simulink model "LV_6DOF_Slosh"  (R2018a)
settings: Solver=FixedStepAuto  StartTime=0.0  StopTime=489.8  FixedStep=0.0002  MaxStep=0.0001  RelTol=2e-6  EnableMultiTasking=on
InitFcn:
  | init
StopFcn:
  | pl
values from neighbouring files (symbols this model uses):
  accel = [97.3083,0,0]    [init.m]
  AcNoise = 0.1    [init.m]
  BBrcs = [82, 0.0, +3.375]    [init.m]
  Cdelay = 0.005    [init.m]
  Cza1 = FCS_Gains_Stg1(:, 5)    [init.m]
  d2r = pi/180    (= 0.0174532925199)    [init.m]    (also in pl.m; LQR_Design.m)
  Euler_0 = [90, 89.98, 0]*d2r    [init.m]
  fairing_mass = 1047.7*kg2slug    (= 71.7904994)    [init.m]
  Ie1 = 28.17    [init.m]
  Ie2 = 258.74    [init.m]
  Islosh = 1    [init.m]
  Isp = 65    [init.m]
  Ixxpr = Mass_Props(:,2)    [init.m]
  Ixypr = Mass_Props(:,5)    [init.m]
  Ixzpr = Mass_Props(:,6)    [init.m]
  Iyypr = Mass_Props(:,3)    [init.m]
  Iyzpr = Mass_Props(:,7)    [init.m]
  Izzpr = Mass_Props(:,4)    [init.m]
  Jdir = zeros(3,nt)    [init.m]
  JJ1 = Commands_2(:,2)    [init.m]
  JJ2 = Commands_2(:,3)    [init.m]
  JJ3 = Commands_2(:,4)    [init.m]
  Jloc = Jdir    [init.m]
  K_estim1 = FCS_Gains_Stg1(:,21)    [init.m]
  Kl_p1 = FCS_Gains_Stg1(:,12)    [init.m]
  Kl_phi1 = FCS_Gains_Stg1(:,11)    [init.m]
  Km_alfa1 = FCS_Gains_Stg1(:, 8)    [init.m]
  Km_alfin = FCS_Gains_Stg1(:,10)    [init.m]
  Km_q1 = FCS_Gains_Stg1(:, 7)    [init.m]
  Km_q2 = FCS_Gains_Stg2(:,5)    [init.m]
  Km_thet1 = FCS_Gains_Stg1(:, 6)    [init.m]
  Km_thet2 = FCS_Gains_Stg2(:,4)    [init.m]
  Km_thin1 = FCS_Gains_Stg1(:, 9)    [init.m]
  Km_thin2 = FCS_Gains_Stg2(:,6)    [init.m]
  Kmix2 = [ 0,   -1,    0;          0,    0,   -1]    [init.m]
  Kml1_1 = ee*FCS_Gains_Stg1(:,18)    [init.m]
  Kml2_1 = ee*FCS_Gains_Stg1(:,19)    [init.m]
  Kml2_2 = ee*FCS_Gains_Stg2(:,10)    [init.m]
  Kn_beta1 = FCS_Gains_Stg1(:,15)    [init.m]
  Kn_betin = FCS_Gains_Stg1(:,17)    [init.m]
  Kn_psi1 = FCS_Gains_Stg1(:,13)    [init.m]
  Kn_psi2 = FCS_Gains_Stg2(:,7)    [init.m]
  Kn_psin1 = FCS_Gains_Stg1(:,16)    [init.m]
  Kn_psin2 = FCS_Gains_Stg2(:,9)    [init.m]
  Kn_r1 = FCS_Gains_Stg1(:,14)    [init.m]
  Kn_r2 = FCS_Gains_Stg2(:,8)    [init.m]
  Le1 = 1.203    [init.m]
  Le2 = 2.892    [init.m]
  Massgn1 = ee*FCS_Gains_Stg1(:,2)    [init.m]
  Massgn2 = ee*FCS_Gains_Stg2(:,2)    [init.m]
  mdot1 = 2.5058    [init.m]
  mdot2 = 2.5058    [init.m]
  me1 = 9.325    [init.m]
  me2 = 13.927    [init.m]
  mrc = [x_ref, y_ref, z_ref]    [init.m]
  Msfue = Slosh(:,3)    [init.m]
  Mslox = Slosh(:,2)    [init.m]
  msspr = Mass_Props(:,1)    [init.m]
  Mvsls = Slosh(:,1)    [init.m]
  post_sep_wait = 4    [init.m]
  pre_sep_wait = 4    [init.m]
  Qbar1 = FCS_Gains_Stg1(:, 4)    [init.m]
  qtc1 = interp1(timi2(1:iend),Commands_2(1:iend, 9),timi2,'linear','extrap')    [init.m]
  qtc2 = interp1(timi2(1:iend),Commands_2(1:iend,10),timi2,'linear','extrap')    [init.m]
  qtc3 = interp1(timi2(1:iend),Commands_2(1:iend,11),timi2,'linear','extrap')    [init.m]
  qtc4 = interp1(timi2(1:iend),Commands_2(1:iend,12),timi2,'linear','extrap')    [init.m]
  r2d = 1/d2r    (= 57.2957795131)    [init.m]    (also in pl.m; LQR_Design.m)
  RBrcs = [82, +3.375, 0.0]    [init.m]
  Rfuel = Slosh(:,11)    [init.m]
  Rlox = Slosh(:,10)    [init.m]
  s1_dry_mass = 445.4969    [init.m]
  s1_init_prop_mass = 3.8002e+03    (= 3800.2)    [init.m]
  s2_dry_mass = 175.9451    [init.m]
  s2_init_prop_mass = 801.7606    [init.m]
  sp = 7.52    [init.m]
  Sref = 44.4146    [init.m]
  stage_to_fairing_sep_time = 34.7    [init.m]
  T3b = 176.6    [init.m]
  TBrcs = [82, 0.0, -3.375]    [init.m]
  thpnd = 15    [init.m]
  timi2 = Commands_2(:,1)    [init.m]
  TqLoad = 1    [init.m]
  tvc10 = [Xgmb2, 0.0,  0.0]    [init.m]
  tvc2 = [Xgmb1,  1.0202,  -2.4638]    [init.m]
  tvc3 = [Xgmb1, -1.0202,  -2.4638]    [init.m]
  tvc4 = [Xgmb1, -2.4638,  -1.0202]    [init.m]
  tvc5 = [Xgmb1, -2.4638,   1.0202]    [init.m]
  tvc6 = [Xgmb1, -1.0202,   2.4638]    [init.m]
  tvc7 = [Xgmb1,  1.0202,   2.4638]    [init.m]
  tvc8 = [Xgmb1,  2.4638,   1.0202]    [init.m]
  tvc9 = [Xgmb1,  0.0,      0.0]    [init.m]
  velpnd = 3    [init.m]
  Vrelgn1 = FCS_Gains_Stg1(:, 3)    [init.m]
  Vrelgn2 = FCS_Gains_Stg2(:,3)    [init.m]
  W_lowp1 = FCS_Gains_Stg1(:,22)    [init.m]
  W_nfilt1 = FCS_Gains_Stg1(:,20)    [init.m]
  Xcgpr = Mass_Props(:,8)    [init.m]
  Xfuel = Slosh(:,9)    [init.m]
  Xgmb1 = 10.7062    [init.m]
  Xgmb2 = 82.538    [init.m]
  Xlox = Slosh(:,8)    [init.m]
  Ycgpr = Mass_Props(:,9)    [init.m]
  Zcgpr = Mass_Props(:,10)    [init.m]
  Ztfue = Slosh(:,7)    [init.m]
  Ztlox = Slosh(:,6)    [init.m]
undefined symbols (not defined in the file or in its folder): Cl, Cl2, Cm, Cm2, Cn, Cn2, Continuous, cosd, CX, CX2, CY, CY2, CZ, CZ2, Dryden, Earth, F, ft, Isp1, Isp2, km, Kmix1, LBrcs, Light, MIL, q, r, sigbuilder_block, sind, STD, tvc1, WGS84
libraries: sharedutil x28, Actuator_Lib x18, simulink x4, aerolibasang x3, aerolibwind2 x3, sharedtransform x3, aerolibobsolete x2, aerolibconvert2 x2, aerolibatmos2 x1, aerolibadyn x1, aerolibutil x1
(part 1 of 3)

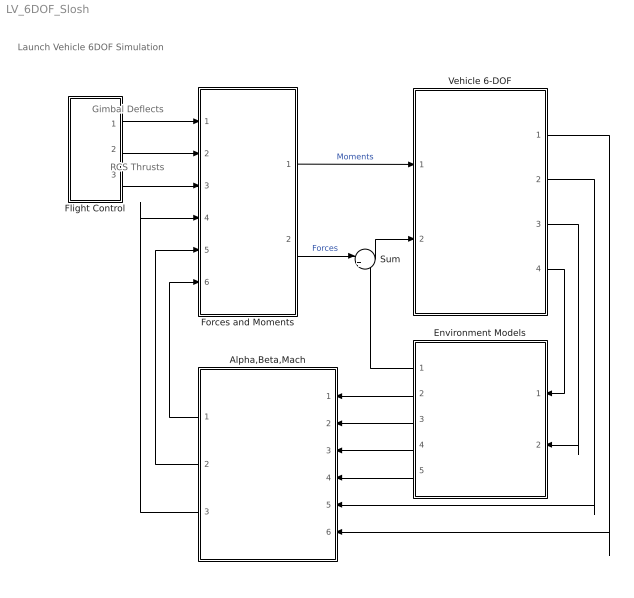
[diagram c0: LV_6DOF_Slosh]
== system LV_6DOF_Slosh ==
  note: Launch Vehicle 6DOF Simulation
  note: Gimbal Deflects
  note: RCS Thrusts
  Alpha,Beta,Mach : Subsystem
  Environment Models : Subsystem
  Flight Control : Subsystem
  Forces and Moments : Subsystem
  Sum : Sum  Inputs=|++
  Vehicle 6-DOF : Subsystem
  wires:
  Vehicle 6-DOF/4(Ve) -> Environment Models/1(Ve)
  Vehicle 6-DOF/3(Height) -> Environment Models/2(Height)
  Environment Models/2(Speed of Sound) -> Alpha,Beta,Mach/1(Speed of Sound)
  Environment Models/4(Air Density) -> Alpha,Beta,Mach/3(Air Density)
  Vehicle 6-DOF/2(Vb) -> Alpha,Beta,Mach/5(Vb)
  Vehicle 6-DOF/1(w) -> Alpha,Beta,Mach/6("p,q,r ")
  Sum/1 -> Vehicle 6-DOF/2(Fxyz)
  Forces and Moments/2(X,Y,Z) -> Sum/1  "Forces"
  Environment Models/1(Fgrv) -> Sum/2
  Forces and Moments/1(LMN) -> Vehicle 6-DOF/1(Mxyz)  "Moments"
  Alpha,Beta,Mach/1(Qbar) -> Forces and Moments/6(Qbar)
  Alpha,Beta,Mach/2(Mach) -> Forces and Moments/5(Mach)
  Alpha,Beta,Mach/3(Incid) -> Forces and Moments/4(Incid)
  Flight Control/1(DY) -> Forces and Moments/1(DY)
  Flight Control/2(DZ) -> Forces and Moments/2(DZ)
  Environment Models/3(Wind Velocity) -> Alpha,Beta,Mach/2(Wind Velocity)
  Environment Models/5(Wind Angular Rates) -> Alpha,Beta,Mach/4(Wind Angular Rates)
  Flight Control/3(Thrcs) -> Forces and Moments/3(Frcs)

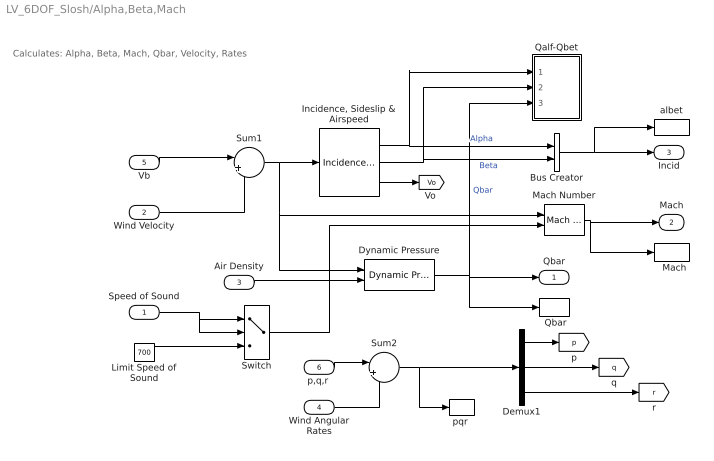
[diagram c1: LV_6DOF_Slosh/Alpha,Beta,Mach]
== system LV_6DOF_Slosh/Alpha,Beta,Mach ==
  note: Calculates: Alpha, Beta, Mach, Qbar, Velocity, Rates
  Speed of Sound : Inport
  Wind Velocity : Inport  Port=2  PortDimensions=3
  Air Density : Inport  Port=3
  Wind Angular Rates : Inport  Port=4  PortDimensions=3
  Vb : Inport  Port=5  PortDimensions=3
  "p,q,r " : Inport  Port=6  PortDimensions=3
  "  Mach" : ToWorkspace  VariableName=Mach  SampleTime=-1
  " Qbar" : ToWorkspace  VariableName=Qbar  SampleTime=-1
  Bus Creator : BusCreator  Inputs=2
  Demux1 : Demux  Outputs=3
  Dynamic Pressure : aerolibasang/Dynamic Pressure
  "Incidence, Sideslip & Airspeed" : aerolibasang/Incidence, Sideslip, & Airspeed
  Limit Speed of Sound : Constant  Value=700
  Mach Number : aerolibasang/Mach Number
  Qalf-Qbet : Subsystem
  Sum1 : Sum  Inputs=|+-
  Sum2 : Sum  Inputs=|++
  Switch : Switch  Threshold=700
  albet : ToWorkspace  VariableName=albet  SampleTime=-1
  "pqr " : ToWorkspace  VariableName=pqr  SampleTime=-1
  Qbar : Outport  InitialOutput=0
  Mach : Outport  Port=2
  Incid : Outport  Port=3
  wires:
  Limit Speed of Sound/1 -> Switch/3
  Switch/1 -> Mach Number/2
  Air Density/1 -> Dynamic Pressure/2
  Demux1/1 -> [p]
  Demux1/3 -> [r]
  Demux1/2 -> [q]
  Sum2/1 -> "pqr "/1, Demux1/1
  "p,q,r "/1 -> Sum2/1
  "Incidence, Sideslip & Airspeed"/1 -> Qalf-Qbet/1(alf), Bus Creator/1  "Alpha"
  Bus Creator/1 -> albet/1, Incid/1
  "Incidence, Sideslip & Airspeed"/2 -> Qalf-Qbet/2(bet), Bus Creator/2  "Beta"
  Speed of Sound/1 -> Switch/2, Switch/1
  Vb/1 -> Sum1/1
  Sum1/1 -> "Incidence, Sideslip & Airspeed"/1, Mach Number/1, Dynamic Pressure/1
  Mach Number/1 -> Mach/1, "  Mach"/1
  Dynamic Pressure/1 -> Qalf-Qbet/3(Qbar), " Qbar"/1, Qbar/1  "Qbar"
  "Incidence, Sideslip & Airspeed"/3 -> [Vo]
  Wind Velocity/1 -> Sum1/2
  Wind Angular Rates/1 -> Sum2/2

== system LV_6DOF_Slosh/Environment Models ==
  note: Gravity Forces in Body (Fx, Fy, Fz)
  note: Environment Models
  note: Geodetic to Body Direction Cosine Matrix
  note: Vehicle Position (Longitude, Latitude, Altitude)
  note: Velocity Relative to Earth
  Ve : Inport
  Height : Inport  Port=2
  COESA Atmosphere Model : aerolibatmos2/COESA Atmosphere Model  units=English (Velocity in ft/s)  spec=MIL-STD-210C  model=Profile  profile_var=Low density  profile_percent=1%  profile_alt=5 km (16404 ft)  envelope_var=High temperature  envelope_percent=1%  action=Warning
  Commands : Subsystem  Tag=STV Subsys  LoadFcn=sigbuilder_block('load');  StartFcn=sigbuilder_block('start');  StopFcn=sigbuilder_block('stop');  ClipboardFcn=sigbuilder_block('clipboard');  mask(Sigbuilder block){tuvar=[0:10]}
      mask help: Sigbuilder GUI
      mask init:
      | if ~strcmp(get_param(bdroot(gcbh),'SimulationStatus'),'stopped') tuvar = sigbuilder_block('maskInit'); end
  Demux2 : Demux  Outputs=3
  Fz1 : Product
  Inertial to Body : Product  Multiplication=Matrix(*)
  Reshape : Reshape
  Terminator1 : Terminator
  "WGS84 Gravity Model " : aerolibobsolete/WGS84 Gravity Model   model=WGS84 Taylor Series  units=English  no_atmos=on  precessing=on  jd_loc=off  month=October  day=10  year=2004  no_centrifugal=on  action=None
  Wind Models : Subsystem
  alti : ToWorkspace  VariableName=alti  SampleTime=-1
  latitude : ToWorkspace  VariableName=latit  SampleTime=-1
  latitude1 : ToWorkspace  VariableName=latit2  SampleTime=-1
  longitud2 : ToWorkspace  VariableName=long2  SampleTime=-1
  longitude : ToWorkspace  VariableName=long  SampleTime=-1
  Fgrv : Outport  InitialOutput=0
  Speed of Sound : Outport  Port=2  InitialOutput=0
  Wind Velocity : Outport  Port=3  InitialOutput=0
  Air Density : Outport  Port=4  InitialOutput=0
  Wind Angular Rates : Outport  Port=5  InitialOutput=0
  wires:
  COESA Atmosphere Model/3 -> [atm]
  Wind Models/2(pg,qg,rg) -> Wind Angular Rates/1
  Wind Models/1(ug,vg,wg) -> Wind Velocity/1
  Ve/1 -> Wind Models/1(Ve)
  COESA Atmosphere Model/4 -> Air Density/1
  COESA Atmosphere Model/1 -> Terminator1/1
  COESA Atmosphere Model/2 -> Speed of Sound/1
  Demux2/2 -> longitude/1
  Demux2/1 -> latitude/1
  Reshape/1 -> Inertial to Body/2
  "WGS84 Gravity Model "/1 -> [ge], Fz1/1
  Fz1/1 -> Reshape/1
  [DCM] -> Inertial to Body/1, Wind Models/3(DCM)
  Inertial to Body/1 -> Fgrv/1
  [mass] -> Fz1/2
  Demux2/3 -> alti/1, COESA Atmosphere Model/1, Wind Models/2(Altitude)  "Altitude"
  Height/1 -> Demux2/1, "WGS84 Gravity Model "/1
  Commands/2(Latitude) -> latitude1/1
  Commands/1(Longitude) -> longitud2/1

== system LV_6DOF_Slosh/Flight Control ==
  note: Flight Control System
  note: Mixing Logic TVC Matrix
  note: Quaternion Error and Guidance Commands
  note: RCS Thrusts (8)
  20ms : TransportDelay  DelayTime=Cdelay  PadeOrder=1
  "20ms " : TransportDelay  DelayTime=Cdelay  PadeOrder=1
  Combine Gimb Accels : Subsystem
  Combine Gimb Deflects : Subsystem
  Combine Shaft Extensions : Subsystem
  Commands : Subsystem
  Demux : Demux  Outputs=[8,8]
  Gain : Gain  Gain=Kmix1  Multiplication=Matrix(K*u) (u vector)
  Gain1 : Gain  Gain=Kmix2  Multiplication=Matrix(K*u) (u vector)
  Lateral FCS : Subsystem
  Mux : Mux  Inputs=3
  Pitch FCS : Subsystem
  "RCS " : ToWorkspace  VariableName=RCS  SampleTime=-1
  RCS Control : Subsystem
  Stage-1 Non-Linear Actuators : Subsystem
  Stage-2 Non-Linear Actuators : Subsystem
  DY : Outport
  DZ : Outport  Port=2
  Thrcs : Outport  Port=3
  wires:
  Pitch FCS/1(DQ_tvc) -> Mux/2
  Lateral FCS/1(DP_tvc) -> Mux/1
  Lateral FCS/2(DR_tvc) -> Mux/3
  Mux/1 -> "20ms "/1
  Gain1/1 -> Stage-2 Non-Linear Actuators/1(act_cmd)
  Gain/1 -> Stage-1 Non-Linear Actuators/1(act_cmd)
  Demux/1 -> Pitch FCS/1(dy)  "dy"
  Demux/2 -> Lateral FCS/3(dz)  "dz"
  Commands/3(Thet_err) -> RCS Control/1(The_err), Pitch FCS/2(Thet_err)
  Commands/2(Phi_err) -> RCS Control/2(Phi_err), Lateral FCS/1(Phi_err)
  Commands/1(Psi_err) -> RCS Control/3(Psi_err), Lateral FCS/2(Psi_err)
  RCS Control/1(f(i)) -> 20ms/1
  Stage-1 Non-Linear Actuators/1(delta) -> Combine Gimb Deflects/2(del(1:8)), Demux/1
  Combine Gimb Deflects/1(DY) -> DY/1
  Combine Gimb Deflects/2(DZ) -> DZ/1
  Stage-2 Non-Linear Actuators/1(delta) -> Combine Gimb Deflects/1(del9)
  Stage-2 Non-Linear Actuators/2(deldd) -> Combine Gimb Accels/1(deldd9)
  Stage-1 Non-Linear Actuators/2(deldd) -> Combine Gimb Accels/2(deldd(1:8))
  "20ms "/1 -> Gain1/1, Gain/1
  20ms/1 -> "RCS "/1, Thrcs/1
  Stage-1 Non-Linear Actuators/3(Xpyz) -> Combine Shaft Extensions/2(Xp(1:8))
  Stage-2 Non-Linear Actuators/3(Xpyz) -> Combine Shaft Extensions/1(Xp9)

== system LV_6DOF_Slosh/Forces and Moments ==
  note: Moments and Forces due to Aero, Engine and RCS Thrusts
  note: Total Forces
  note: Measured Body CG Accelerat
  note: Total Moments
  note: Lift Forward Side-Force
  note: Slosh Dynamics
  DY : Inport
  DZ : Inport  Port=2
  Frcs : Inport  Port=3
  Incid : Inport  Port=4
  Mach : Inport  Port=5
  Qbar : Inport  Port=6
  Aero Forces : Subsystem
  Axyz : ToWorkspace  VariableName=Axyz  SampleTime=-1
  Divide : Product  Inputs=*/
  Forces : Subsystem
  Invert 3x3 Matrix : aerolibutil/Invert  3x3 Matrix
  Propulsion : Subsystem
  Slosh Forces/Torques : Subsystem
  Sum : Sum  Inputs=+++
  Sum1 : Sum  Inputs=+++
  body 2 NED Transform : Product  Multiplication=Matrix(*)
  LMN : Outport  InitialOutput=0
  X,Y,Z : Outport  Port=2  InitialOutput=0
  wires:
  Sum/1 -> LMN/1
  Divide/1 -> Axyz/1, [Axyz]
  Sum1/1 -> X,Y,Z/1, Divide/1, body 2 NED Transform/2
  [mass] -> Divide/2
  Invert 3x3 Matrix/1 -> body 2 NED Transform/1
  [DCM] -> Invert 3x3 Matrix/1
  Incid/1 -> Aero Forces/1(Incid)
  Mach/1 -> Aero Forces/2(Mach)
  Qbar/1 -> Aero Forces/3(qbar)
  Aero Forces/1(Faero) -> Sum1/2
  Aero Forces/2(Maero) -> Sum/2
  Frcs/1 -> Propulsion/1(Frcs)
  DY/1 -> Propulsion/2(DY)
  DZ/1 -> Propulsion/3(DZ)
  Propulsion/1(Feng) -> Sum1/1
  Propulsion/2(Teng) -> Sum/1
  body 2 NED Transform/1 -> Forces/1(Fned)  "Fned"
  Slosh Forces/Torques/1(Fsl) -> Sum1/3
  Slosh Forces/Torques/2(Tsl) -> Sum/3

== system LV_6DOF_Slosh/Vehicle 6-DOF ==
  note: Flight Path Angle and Direction
  note: Forces and Moments
  note: Launch Vehicle Dynamics
  note: Sensors
  Mxyz : Inport
  Fxyz : Inport  Port=2
  Accelerometer : Subsystem
  Custom Variable Mass 6DoF ECEF (Quaternion) : aerolibobsolete/6DoF ECEF (Quaternion)  units=English (Velocity in ft/s)  mtype=Custom Variable  xg_0=In_Posit  Vm_0=Uvw_0  eul_0=Euler_0  pm_0=pqr_0  mass_0=1.0  mass_e=0.5  mass_f=2.0  inertia=eye(3)  inertia_e=eye(3)  inertia_f=2*eye(3)  ptype=Earth (WGS84)  F=1/298.257223563  R=20925646.3255  w_E=7292115e-11  angle_in=Internal  LG0=0
  Direction : Subsystem
  Gamma : Subsystem
  Idot : Ground
  Mass & Inertias : Subsystem
  Quatern : Subsystem
  Rate Gyros : Subsystem
  Terminator : Terminator
  Terminator1 : Terminator
  Terminator2 : Terminator
  Vbody : ToWorkspace  VariableName=Vb  SampleTime=-1
  ecf 2 geo : Product  Multiplication=Matrix(*)
  mdot : Ground
  quatern : Subsystem
  w : Outport
  Vb : Outport  Port=2
  Height : Outport  Port=3
  Ve : Outport  Port=4
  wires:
  Mass & Inertias/2(Inert) -> Custom Variable Mass 6DoF ECEF (Quaternion)/6
  Mass & Inertias/1(mass) -> Custom Variable Mass 6DoF ECEF (Quaternion)/4
  mdot/1 -> Custom Variable Mass 6DoF ECEF (Quaternion)/3
  Idot/1 -> Custom Variable Mass 6DoF ECEF (Quaternion)/5
  Custom Variable Mass 6DoF ECEF (Quaternion)/1 -> Gamma/1(Vecef), ecf 2 geo/2
  Custom Variable Mass 6DoF ECEF (Quaternion)/3 -> Height/1
  ecf 2 geo/1 -> Direction/1(Ve), Ve/1
  Custom Variable Mass 6DoF ECEF (Quaternion)/8 -> Vb/1, Vbody/1
  Custom Variable Mass 6DoF ECEF (Quaternion)/10 -> Rate Gyros/1(wrb), w/1
  Custom Variable Mass 6DoF ECEF (Quaternion)/6 -> quatern/2(in)
  Custom Variable Mass 6DoF ECEF (Quaternion)/4 -> quatern/1(in1), Quatern/1(in)
  Fxyz/1 -> Custom Variable Mass 6DoF ECEF (Quaternion)/1
  Mxyz/1 -> Custom Variable Mass 6DoF ECEF (Quaternion)/2
  Custom Variable Mass 6DoF ECEF (Quaternion)/2 -> Gamma/2(Recef)
  Custom Variable Mass 6DoF ECEF (Quaternion)/11 -> Accelerometer/1(wdot)
  Custom Variable Mass 6DoF ECEF (Quaternion)/7 -> ecf 2 geo/1
  Custom Variable Mass 6DoF ECEF (Quaternion)/12 -> Terminator/1
  Custom Variable Mass 6DoF ECEF (Quaternion)/5 -> Terminator1/1
  Custom Variable Mass 6DoF ECEF (Quaternion)/9 -> Terminator2/1

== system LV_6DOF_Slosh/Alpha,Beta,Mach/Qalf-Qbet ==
  alf : Inport
  bet : Inport  Port=2
  Qbar : Inport  Port=3
  Mux : Mux  Inputs=2
  Product : Product
  Q_ab : Product
  Qab : ToWorkspace  VariableName=Qab  SampleTime=-1
  "Qalpha " : ToWorkspace  VariableName=Qalfa  SampleTime=-1
  Trigonometric Function : Trigonometry  Operator=cos
  Trigonometric Function1 : Trigonometry  Operator=cos
  Trigonometric Function2 : Trigonometry  Operator=acos
  r2d : Gain  Gain=r2d
  x1 : Product
  x2 : Product
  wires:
  Mux/1 -> "Qalpha "/1
  x2/1 -> Mux/2
  x1/1 -> Mux/1
  Qbar/1 -> Q_ab/2, x1/2, x2/1
  Q_ab/1 -> Qab/1  "Qab"
  Trigonometric Function2/1 -> r2d/1  "ab"
  r2d/1 -> Q_ab/1
  Trigonometric Function/1 -> Product/2
  Product/1 -> Trigonometric Function2/1
  bet/1 -> x2/2, [beta], Trigonometric Function/1
  Trigonometric Function1/1 -> Product/1  "cos(alfa)"
  alf/1 -> x1/1, [alfa], Trigonometric Function1/1

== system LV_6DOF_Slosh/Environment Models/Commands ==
  Demux : Demux  Tag=STV Demux  Outputs=2
  FromWs : FromWorkspace  Tag=STV FromWs  VariableName=tuvar  SampleTime=0
  Longitude : Outport  Tag=STV Outport
  Latitude : Outport  Tag=STV Outport  Port=2
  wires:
  FromWs/1 -> Demux/1
  Demux/1 -> Longitude/1
  Demux/2 -> Latitude/1

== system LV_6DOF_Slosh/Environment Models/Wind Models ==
  note: Air-Speed
  note: Wind Disturbance Model (Shear, Gust, Turbulence)
  Ve : Inport
  Altitude : Inport  Port=2
  DCM : Inport  Port=3
  Discrete Wind Gust Model - On : aerolibwind2/Discrete Wind Gust Model  units=English (Velocity in ft/s)  Gx=on  Gy=on  Gz=on  t_0=20  d_m=[120 120 80]  v_m=[3.5 3.0 3.0]*5
  Dot Product : DotProduct  SaturateOnIntegerOverflow=on
  Dryden Wind Turbulence Model (Continuous (+q -r)) : aerolibwind2/Dryden Wind Turbulence Model  (Continuous (+q -r))  units=English (Velocity in ft/s)  spec=MIL-F-8785C  model=Continuous Dryden (+q -r)  W20=5  Wdeg=-80  TurbProb=10^-2 - Light  L_high=533.4  Wingspan=4  ts=0.1  Seed=[23341 23342 23343 23344]  T_on=on
  Sum : Sum  Inputs=+++
  V : Math  Operator=sqrt
  V0 : ToWorkspace  VariableName=V0  SampleTime=-1
  Wind Shear Model : aerolibwind2/Wind Shear Model  units=English (Velocity in ft/s)  phase=Other  W_20=4  Wdeg=-170
  ug,vg,wg : Outport
  pg,qg,rg : Outport  Port=2
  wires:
  Wind Shear Model/1 -> Sum/1
  Discrete Wind Gust Model - On/1 -> Sum/3
  V/1 -> V0/1, [V0], Discrete Wind Gust Model - On/1, Dryden Wind Turbulence Model (Continuous (+q -r))/2
  Ve/1 -> Dot Product/1, Dot Product/2
  Dot Product/1 -> V/1
  Altitude/1 -> Wind Shear Model/1, Dryden Wind Turbulence Model (Continuous (+q -r))/1
  DCM/1 -> Dryden Wind Turbulence Model (Continuous (+q -r))/3, Wind Shear Model/2
  Dryden Wind Turbulence Model (Continuous (+q -r))/1 -> Sum/2
  Dryden Wind Turbulence Model (Continuous (+q -r))/2 -> pg,qg,rg/1
  Sum/1 -> ug,vg,wg/1

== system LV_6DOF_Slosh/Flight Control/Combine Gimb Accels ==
  note: Pitch Gimbal Accels (8+1)
  note: Yaw Gimbal Accels (8+1)
  deldd9 : Inport
  deldd(1:8) : Inport  Port=2
  Demux : Demux  Outputs=[8,8]
  Demux2 : Demux  Outputs=2
  Ground{,1..3} (4 alike) : Ground
  Memory : Memory
  Memory1 : Memory
  Mux{1..4} (4 alike) : Mux  Inputs=[8,1]
  Switch1 : Switch  Criteria=u2 > Threshold
  Switch2 : Switch  Criteria=u2 > Threshold
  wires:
  deldd(1:8)/1 -> Demux/1
  Demux2/2 -> Mux2/2  "dz9"
  Demux2/1 -> Mux1/2  "dy9"
  deldd9/1 -> Demux2/1
  Demux/2 -> Mux4/1  "dz(1:8)"
  Demux/1 -> Mux3/1  "dy(1:8)"
  Mux3/1 -> Switch2/3
  Ground/1 -> Mux3/2
  Mux1/1 -> Switch2/1
  Ground3/1 -> Mux2/1
  [stage_sep] -> Switch2/2, Switch1/2
  Ground1/1 -> Mux4/2
  Mux4/1 -> Switch1/3
  Mux2/1 -> Switch1/1
  Ground2/1 -> Mux1/1
  Switch2/1 -> Memory/1
  Memory/1 -> [Dyedd]
  Switch1/1 -> Memory1/1
  Memory1/1 -> [Dzedd]

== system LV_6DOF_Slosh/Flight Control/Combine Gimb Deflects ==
  note: Yaw Engine (8+1) Deflections (rad)
  note: Pitch Engine (8+1) Deflections (rad)
  del9 : Inport
  del(1:8) : Inport  Port=2
  "DY " : ToWorkspace  VariableName=DY  SampleTime=-1
  "DZ " : ToWorkspace  VariableName=DZ  SampleTime=-1
  Demux : Demux  Outputs=[8,8]
  Demux2 : Demux  Outputs=2
  Ground{,1..3} (4 alike) : Ground
  Mux{1..4} (4 alike) : Mux  Inputs=[8,1]
  Switch1 : Switch  Criteria=u2 > Threshold
  Switch2 : Switch  Criteria=u2 > Threshold
  DY : Outport
  DZ : Outport  Port=2
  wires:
  Switch2/1 -> DY/1, [Dye], "DY "/1
  Ground2/1 -> Mux1/1
  Mux2/1 -> Switch1/1
  Switch1/1 -> DZ/1, [Dze], "DZ "/1
  Mux4/1 -> Switch1/3
  Ground1/1 -> Mux4/2
  [stage_sep] -> Switch1/2, Switch2/2
  Ground3/1 -> Mux2/1
  Mux1/1 -> Switch2/1
  Ground/1 -> Mux3/2
  Mux3/1 -> Switch2/3
  Demux/1 -> Mux3/1  "dy(1:8)"
  Demux/2 -> Mux4/1  "dz(1:8)"
  del9/1 -> Demux2/1
  Demux2/1 -> Mux1/2  "dy9"
  Demux2/2 -> Mux2/2  "dz9"
  del(1:8)/1 -> Demux/1

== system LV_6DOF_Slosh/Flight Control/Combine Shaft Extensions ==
  note: Pitch Act Shaft Extensions (8+1)
  note: Yaw Act Shaft Extensions (8+1)
  note: Shaft Position Combine
  Xp9 : Inport
  Xp(1:8) : Inport  Port=2
  Demux : Demux  Outputs=[8,8]
  Demux2 : Demux  Outputs=2
  Ground{,1..3} (4 alike) : Ground
  Mux{1..4} (4 alike) : Mux  Inputs=[8,1]
  Switch1 : Switch  Criteria=u2 > Threshold
  Switch2 : Switch  Criteria=u2 > Threshold
  "Xpy " : ToWorkspace  VariableName=Xpy  SampleTime=-1
  Xpz : ToWorkspace  VariableName=Xpz  SampleTime=-1
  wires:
  Xp(1:8)/1 -> Demux/1
  Demux2/2 -> Mux2/2  "Xpz9"
  Demux2/1 -> Mux1/2  "Xpy9"
  Xp9/1 -> Demux2/1
  Demux/2 -> Mux4/1  "Xpz(1:8)"
  Demux/1 -> Mux3/1  "Xpy(1:8)"
  Mux3/1 -> Switch2/3
  Ground/1 -> Mux3/2
  Mux1/1 -> Switch2/1
  Ground3/1 -> Mux2/1
  [stage_sep] -> Switch2/2, Switch1/2
  Ground1/1 -> Mux4/2
  Mux4/1 -> Switch1/3
  Mux2/1 -> Switch1/1
  Ground2/1 -> Mux1/1
  Switch2/1 -> "Xpy "/1
  Switch1/1 -> Xpz/1

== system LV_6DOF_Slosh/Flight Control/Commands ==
  note: Pad to Body Quaternion fbk
  note: Flight Control Commands
  note: Guidance
  AM/ Inclination : Subsystem
  Demux2 : Demux  Outputs=3
  ECEF to ECI : Subsystem
  Quaternion Command : Subsystem
  Quaternion Error Function : MATLAB Function  TreatAsAtomicUnit=on
  Quaterr : ToWorkspace  VariableName=Qer  SampleTime=-1
  Sum2 : Sum  Inputs=|++
  Psi_err : Outport
  Phi_err : Outport  Port=2
  Thet_err : Outport  Port=3
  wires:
  [qtb3] -> Quaternion Error Function/2(qb)
  Quaternion Error Function/1(qfb) -> Demux2/1, Quaterr/1
  Demux2/1 -> Phi_err/1
  ECEF to ECI/2(Veci) -> AM/ Inclination/2(Veci)
  [Recef] -> ECEF to ECI/1(Recef)
  [Vecef] -> ECEF to ECI/2(Vecef)
  ECEF to ECI/1(Reci) -> AM/ Inclination/1(Reci)
  Sum2/1 -> Psi_err/1
  AM/ Inclination/1(dyaw) -> Sum2/2
  Demux2/3 -> Sum2/1
  Quaternion Command/1(Quatin) -> Quaternion Error Function/1(qc)
  Demux2/2 -> Thet_err/1

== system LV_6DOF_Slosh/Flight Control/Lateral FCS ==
  note: Lateral Flight Control System
  Phi_err : Inport
  Psi_err : Inport  Port=2
  dz : Inport  Port=3
  First Stage FCS : Subsystem
  Second Stage FCS : Subsystem
  Sum : Sum  Inputs=|++
  DP_tvc : Outport
  DR_tvc : Outport  Port=2
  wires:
  Phi_err/1 -> First Stage FCS/1(Phi_err)
  Psi_err/1 -> Second Stage FCS/1(Psi_err), First Stage FCS/2(Psi_err)
  First Stage FCS/1(DP_tvc) -> DP_tvc/1
  Sum/1 -> DR_tvc/1
  First Stage FCS/2(DR_tvc) -> Sum/1
  Second Stage FCS/1(DR_tvc) -> Sum/2
  dz/1 -> First Stage FCS/3(dz)  "(rad)"

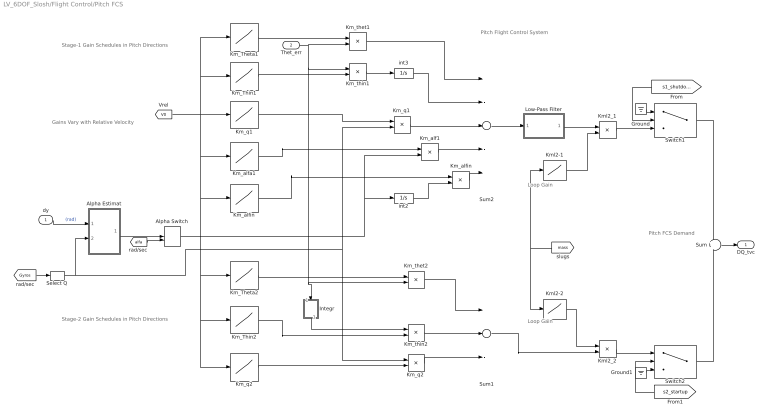
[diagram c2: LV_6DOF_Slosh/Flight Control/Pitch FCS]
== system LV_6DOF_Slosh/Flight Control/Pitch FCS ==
  note: Stage-1 Gain Schedules in Pitch Directions
  note: Pitch Flight Control System
  note: Stage-2 Gain Schedules in Pitch Directions
  note: Pitch FCS Demand
  note: Loop Gain
  note: Loop Gain
  note: Gains Vary with Relative Velocity
  dy : Inport
  Thet_err : Inport  Port=2
  " Km_alfin" : Product
  Alpha Estimat : Subsystem
  Alpha Switch : ManualSwitch
  Ground : Ground
  Ground1 : Ground
  Integr : Subsystem
  Km_Theta1 : Lookup  InputValues=Vrelgn1  Table=Km_thet1
  Km_Theta2 : Lookup  InputValues=Vrelgn2  Table=Km_thet2
  Km_Thin1 : Lookup  InputValues=Vrelgn1  Table=Km_thin1
  Km_Thin2 : Lookup  InputValues=Vrelgn2  Table=Km_thin2
  Km_alf1 : Product
  Km_alfa1 : Lookup  InputValues=Vrelgn1  Table=Km_alfa1
  Km_alfin : Lookup  InputValues=Vrelgn1  Table=Km_alfin
  Km_q1 : Lookup  InputValues=Vrelgn1  Table=Km_q1
  "Km_q1 " : Product
  Km_q2 : Lookup  InputValues=Vrelgn2  Table=Km_q2
  "Km_q2 " : Product
  Km_thet1 : Product
  Km_thet2 : Product
  Km_thin1 : Product
  Km_thin2 : Product
  Kml2-1 : Lookup  InputValues=Massgn1  Table=Kml2_1
  Kml2-2 : Lookup  InputValues=Massgn2  Table=Kml2_2
  Kml2_1 : Product
  Kml2_2 : Product
  Low-Pass Filter : Subsystem
  Select Q : Selector  InputPortWidth=3  IndexOptions=Index vector (dialog)  Indices=[2]  OutputSizes=1
  Sum : Sum  Inputs=+|+
  Sum1 : Sum  Inputs=---
  Sum2 : Sum  Inputs=-----
  Switch1 : Switch  Criteria=u2 > Threshold
  Switch2 : Switch  Criteria=u2 > Threshold
  int2 : Integrator
  int3 : Integrator
  DQ_tvc : Outport
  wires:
  Km_alf1/1 -> Sum2/4
  "Km_q1 "/1 -> Sum2/3
  Km_thet1/1 -> Sum2/1
  Select Q/1 -> "Km_q1 "/2, "Km_q2 "/1, Alpha Estimat/2(q)
  Kml2-1/1 -> Kml2_1/2
  Km_thet2/1 -> Sum1/1
  "Km_q2 "/1 -> Sum1/3
  [V0] -> Km_q2/1, Km_Thin2/1, Km_Theta2/1, Km_alfin/1, Km_alfa1/1, Km_Theta1/1, Km_Thin1/1, Km_q1/1
  [mass] -> Kml2-2/1, Kml2-1/1
  [Gyros] -> Select Q/1
  Ground/1 -> Switch1/1
  Kml2_1/1 -> Switch1/3
  Kml2_2/1 -> Switch2/1
  Sum1/1 -> Kml2_2/2
  Ground1/1 -> Switch2/3
  Switch2/1 -> Sum/2
  Switch1/1 -> Sum/1
  Sum/1 -> DQ_tvc/1
  " Km_alfin"/1 -> Sum2/5
  int2/1 -> " Km_alfin"/2
  dy/1 -> Alpha Estimat/1(dy)  "(rad)"
  [alfa] -> Alpha Switch/2
  Alpha Switch/1 -> Km_alf1/2, int2/1
  Alpha Estimat/1(alfest) -> Alpha Switch/1
  Thet_err/1 -> Integr/1(in), Km_thet2/2, Km_thin1/1, Km_thet1/2
  Km_thin2/1 -> Sum1/2
  [s1_shutdown] -> Switch1/2
  [s2_startup] -> Switch2/2
  Km_q2/1 -> "Km_q2 "/2
  Kml2-2/1 -> Kml2_2/1
  Integr/1(ou) -> Km_thin2/1
  Km_Theta2/1 -> Km_thet2/1
  Km_Thin2/1 -> Km_thin2/2
  Sum2/1 -> Low-Pass Filter/1(u)
  Low-Pass Filter/1(y) -> Kml2_1/1
  Km_thin1/1 -> int3/1
  int3/1 -> Sum2/2
  Km_Theta1/1 -> Km_thet1/1
  Km_Thin1/1 -> Km_thin1/2
  Km_q1/1 -> "Km_q1 "/1
  Km_alfa1/1 -> Km_alf1/1
  Km_alfin/1 -> " Km_alfin"/1

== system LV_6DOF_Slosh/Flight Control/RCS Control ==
  note: Pitch and Yaw RCS is: after Staging and before S2 Ignition after MECO
  note: Activate RCS Control after Stg1 MECO
  note: RCS Phase-Plane Logic
  note: Roll RCS begins after Stg2 Ignition
  The_err : Inport
  Phi_err : Inport  Port=2
  Psi_err : Inport  Port=3
  Mux : Mux  Inputs=3
  Mux1 : Mux  Inputs=3
  Phase-Plane Controller : Subsystem
  Select P : Selector  InputPortWidth=3  IndexOptions=Index vector (dialog)  Indices=[1]  OutputSizes=1
  Select Q : Selector  InputPortWidth=3  IndexOptions=Index vector (dialog)  Indices=[2]  OutputSizes=1
  Select R : Selector  InputPortWidth=3  IndexOptions=Index vector (dialog)  Indices=[3]  OutputSizes=1
  coast switch1 : Subsystem
  coast switch2 : Subsystem
  coast switch3 : Subsystem
  coast switch4 : Subsystem
  stage-sep switch : Subsystem
  f(i) : Outport
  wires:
  Psi_err/1 -> coast switch4/1(in)
  Select R/1 -> coast switch2/1(in)
  Phi_err/1 -> Mux/1
  Select P/1 -> Mux1/1
  Phase-Plane Controller/1(f(i)) -> stage-sep switch/1(in)
  Mux/1 -> Phase-Plane Controller/2(atter)
  Mux1/1 -> Phase-Plane Controller/1(rater)
  [Gyros] -> Select R/1, Select Q/1, Select P/1
  stage-sep switch/1(ou) -> f(i)/1
  Select Q/1 -> coast switch1/1(in)
  The_err/1 -> coast switch3/1(in)
  coast switch1/1(ou) -> Mux1/2
  coast switch2/1(ou) -> Mux1/3
  coast switch3/1(ou) -> Mux/2
  coast switch4/1(ou) -> Mux/3

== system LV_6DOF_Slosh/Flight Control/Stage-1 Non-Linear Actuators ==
  note: Gimbal Deflections (rad)
  note: Gimbal Deflect Command (rad)
  note: Actuator Power (Watt)
  note: Engine Rotat. Accelerat. (rad/sec^2)
  note: Actuator Shaft Extension (ft)
  act_cmd : Inport
  Demux1 : Demux  Outputs=[8,8]
  Load-Torque : Subsystem
  Memory : Memory
  Mux1 : Mux  Inputs=[8,8]
  Mux2 : Mux  Inputs=[8,8]
  Mux5 : Mux  Inputs=[8,8]
  "Power " : ToWorkspace  VariableName=Power  SampleTime=-1
  Stage-1 Pitch Non-Linear Actuators : Subsystem
  Stage-1 Yaw Non-Linear Actuators : Subsystem
  Sum : Sum  Inputs=++|
  Sum1 : Sum  Inputs=++|
  Switch1 : Switch  Criteria=u2 > Threshold
  delta : Outport
  deldd : Outport  Port=2
  Xpyz : Outport  Port=3
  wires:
  [s1_shutdown] -> Switch1/2
  Switch1/1 -> Demux1/1, Memory/1
  act_cmd/1 -> Switch1/3
  Memory/1 -> Switch1/1
  Demux1/1 -> Stage-1 Pitch Non-Linear Actuators/1(Dy_cmd)  "dy"
  Demux1/2 -> Stage-1 Yaw Non-Linear Actuators/1(Dz_cmd)  "dz"
  Stage-1 Yaw Non-Linear Actuators/2(Dz_pow) -> Sum/2
  Sum1/1 -> "Power "/1
  Stage-1 Pitch Non-Linear Actuators/2(Dy_pow) -> Sum/1
  Mux5/1 -> delta/1
  Stage-1 Yaw Non-Linear Actuators/3(Dz_dd) -> Mux1/2
  Stage-1 Pitch Non-Linear Actuators/3(Dy_dd) -> Mux1/1
  Stage-1 Pitch Non-Linear Actuators/1(Dy_out) -> Mux5/1
  Stage-1 Yaw Non-Linear Actuators/1(Dz_out) -> Mux5/2
  Mux1/1 -> deldd/1
  Sum/1 -> Sum1/2
  [Pow2] -> Sum1/1
  Stage-1 Pitch Non-Linear Actuators/4(Xpy) -> Mux2/1
  Stage-1 Yaw Non-Linear Actuators/4(Xpz) -> Mux2/2
  Mux2/1 -> Xpyz/1
  Load-Torque/1(TLy) -> Stage-1 Pitch Non-Linear Actuators/2(Ty_Load)
  Load-Torque/2(TLz) -> Stage-1 Yaw Non-Linear Actuators/2(Tz_Load)

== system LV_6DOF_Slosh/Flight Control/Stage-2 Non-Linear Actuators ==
  note: Act Position Measurem Noise
  note: Gimbal Deflect Command (rad)
  note: Gimbal Deflections (rad)
  note: Engine Rotat. Accelerat. (rad/sec^2)
  note: Actuator Shaft Extension (ft)
  act_cmd : Inport
  Demux1 : Demux  Outputs=[1,1]
  Demux2 : Demux  Outputs=[1,1]
  Ground3 : Ground
  Load-Torque : Subsystem
  Measurem Error 0.1 (deg) : UniformRandomNumber  Minimum=-[1, 1]*AcNoise*d2r  Maximum=[1, 1]*AcNoise*d2r  Seed=[10,20]  SampleTime=0.01
  Mux1 : Mux  Inputs=[1,1]
  Mux2 : Mux  Inputs=[1,1]
  Mux5 : Mux  Inputs=[1,1]
  Pitch Actuator : Actuator_Lib/Stage2 Actuator
  RT : RateTransition  OutPortSampleTime=0.0002
  Sum : Sum  Inputs=++|
  Switch1 : Switch  Criteria=u2 > Threshold
  Switch2 : Switch  Criteria=u2 > Threshold
  Yaw Actuator : Actuator_Lib/Stage2 Actuator
  delta : Outport
  deldd : Outport  Port=2
  Xpyz : Outport  Port=3
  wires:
  Demux1/1 -> Pitch Actuator/1  "dy9"
  Demux1/2 -> Yaw Actuator/1  "dz9"
  Switch1/1 -> Demux1/1
  act_cmd/1 -> Switch1/1
  Ground3/1 -> Switch2/3, Switch1/3
  Pitch Actuator/1 -> Mux5/1  "dy"
  Yaw Actuator/1 -> Mux5/2  "dz"
  Demux2/1 -> Pitch Actuator/2
  Demux2/2 -> Yaw Actuator/2
  Measurem Error 0.1 (deg)/1 -> RT/1
  [s2_startup] -> Switch1/2, Switch2/2
  Pitch Actuator/2 -> Sum/1
  Yaw Actuator/2 -> Sum/2
  Sum/1 -> [Pow2]
  Yaw Actuator/3 -> Mux1/2  "dzdd"
  Pitch Actuator/3 -> Mux1/1  "dydd"
  Mux5/1 -> delta/1
  Mux1/1 -> deldd/1
  Yaw Actuator/4 -> Mux2/2  "Xpz"
  Pitch Actuator/4 -> Mux2/1  "Xpy"
  Mux2/1 -> Xpyz/1
  RT/1 -> Switch2/1
  Load-Torque/2(TLz) -> Yaw Actuator/3
  Load-Torque/1(TLy) -> Pitch Actuator/3
  Switch2/1 -> Demux2/1

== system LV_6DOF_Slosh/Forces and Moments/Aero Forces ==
  note: Dynamic Pressure
  note: Aero coefficients (CX,CY,CZ,Cl,Cm,Cn)
  Incid : Inport
  Mach : Inport  Port=2
  qbar : Inport  Port=3
  "Aerodynamic Forces and Moments (Fx,Fy,Fz), (Lx,My,Nz)" : aerolibadyn/Aerodynamic Forces and Moments   inputAxes=Body  outputForceAxes=Body  outputMomentAxes=Body  S=Sref  b=sp  cbar=ch
  Moments Reference Center (MRC) in (feet) : Constant  Value=mrc
  Stage-1 Aerodynamic Coefficients : Subsystem
  Stage-2 Aerodynamic Coefficients : Subsystem
  Switch3 : Switch  Criteria=u2 > Threshold
  Faero : Outport
  Maero : Outport  Port=2
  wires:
  Mach/1 -> Stage-2 Aerodynamic Coefficients/2(Mach), Stage-1 Aerodynamic Coefficients/2(Mach)
  Incid/1 -> Stage-2 Aerodynamic Coefficients/1(Incid), Stage-1 Aerodynamic Coefficients/1(Incid)
  Moments Reference Center (MRC) in (feet)/1 -> "Aerodynamic Forces and Moments (Fx,Fy,Fz), (Lx,My,Nz)"/4
  [CG] -> "Aerodynamic Forces and Moments (Fx,Fy,Fz), (Lx,My,Nz)"/3
  "Aerodynamic Forces and Moments (Fx,Fy,Fz), (Lx,My,Nz)"/2 -> Maero/1
  "Aerodynamic Forces and Moments (Fx,Fy,Fz), (Lx,My,Nz)"/1 -> Faero/1
  qbar/1 -> "Aerodynamic Forces and Moments (Fx,Fy,Fz), (Lx,My,Nz)"/2
  Stage-2 Aerodynamic Coefficients/1(Coeff) -> Switch3/1
  Stage-1 Aerodynamic Coefficients/1(Coeff) -> Switch3/3
  [stage_sep] -> Switch3/2
  Switch3/1 -> "Aerodynamic Forces and Moments (Fx,Fy,Fz), (Lx,My,Nz)"/1

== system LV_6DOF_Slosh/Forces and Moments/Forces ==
  note: Lift, Forward, and Side Forces
  note: Heading Direction
  Fned : Inport
  Demux : Demux  Outputs=3
  Fe cos y : Product
  Fe sin y : Product
  Fn cos y : Product
  Fn sin y : Product
  Forces : ToWorkspace  VariableName=Flds  SampleTime=-1
  Mux : Mux  Inputs=3
  Sum : Sum  Inputs=|++
  Sum1 : Sum  Inputs=|-+
  cos : Trigonometry  Operator=cos
  sin : Trigonometry
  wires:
  [direct] -> cos/1, sin/1
  Fned/1 -> Demux/1
  Demux/3 -> Mux/1  "FU"
  cos/1 -> Fe cos y/2, Fn cos y/2
  Demux/1 -> Fn sin y/1, Fn cos y/1  "FNorth"
  sin/1 -> Fn sin y/2, Fe sin y/2
  Demux/2 -> Fe cos y/1, Fe sin y/1  "FEast"
  Fe sin y/1 -> Sum/1
  Fn cos y/1 -> Sum/2
  Sum/1 -> Mux/2  "FF"
  Fn sin y/1 -> Sum1/1
  Fe cos y/1 -> Sum1/2
  Sum1/1 -> Mux/3  "FT"
  Mux/1 -> Forces/1

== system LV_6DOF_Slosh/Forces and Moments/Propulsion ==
  note: Gimbal Deflections (rad)
  note: RCS Thrusts (1:8)
  note: Engine Thrusts Versus Time
  note: Propulsion Forces and Torques
  note: Stage-1 Gimbals
  note: Stage-2 Gimbals
  Frcs : Inport
  DY : Inport  Port=2
  DZ : Inport  Port=3
  Dye(1:8) : Selector  InputPortWidth=9  IndexOptions=Index vector (dialog)  Indices=[1:8]  OutputSizes=1
  Dye9 : Selector  InputPortWidth=9  IndexOptions=Index vector (dialog)  Indices=[9]  OutputSizes=1
  Dze(1:8) : Selector  InputPortWidth=9  IndexOptions=Index vector (dialog)  Indices=[1:8]  OutputSizes=1
  Dze9 : Selector  InputPortWidth=9  IndexOptions=Index vector (dialog)  Indices=[9]  OutputSizes=1
  Engine Thrusts : Subsystem
  RCS Jets : Subsystem
  Stage-1 Engine Forces & Torques : Subsystem
  Stage-2 Engine : Subsystem
  Sum1 : Sum  Inputs=|++
  Sum2 : Sum  Inputs=|++
  Switch1 : Switch  Criteria=u2 > Threshold
  Switch3 : Switch  Criteria=u2 > Threshold
  Feng : Outport
  Teng : Outport  Port=2
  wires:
  Engine Thrusts/1(Thrust-1) -> Stage-1 Engine Forces & Torques/1(Thrst1)
  Dze9/1 -> Stage-2 Engine/3(dz)
  DY/1 -> Dye9/1, Dye(1:8)/1
  Dye9/1 -> Stage-2 Engine/2(dy)
  DZ/1 -> Dze9/1, Dze(1:8)/1
  Dye(1:8)/1 -> Stage-1 Engine Forces & Torques/2(DY (rad))
  Dze(1:8)/1 -> Stage-1 Engine Forces & Torques/3(DZ (rad))
  Switch3/1 -> Feng/1
  Stage-1 Engine Forces & Torques/1(Force) -> Switch3/3
  Stage-1 Engine Forces & Torques/2(Torqu) -> Switch1/3
  Frcs/1 -> RCS Jets/1(RCS Jets)
  Stage-2 Engine/1(F10) -> Sum1/1
  RCS Jets/1(Frcs) -> Sum1/2
  Sum1/1 -> Switch3/1
  Stage-2 Engine/2(M10) -> Sum2/1
  RCS Jets/2(Trcs) -> Sum2/2
  Sum2/1 -> Switch1/1
  [s1_shutdown] -> Switch1/2, Switch3/2
  Engine Thrusts/2(Thrust-2) -> Stage-2 Engine/1(Thrst2)
  Switch1/1 -> Teng/1

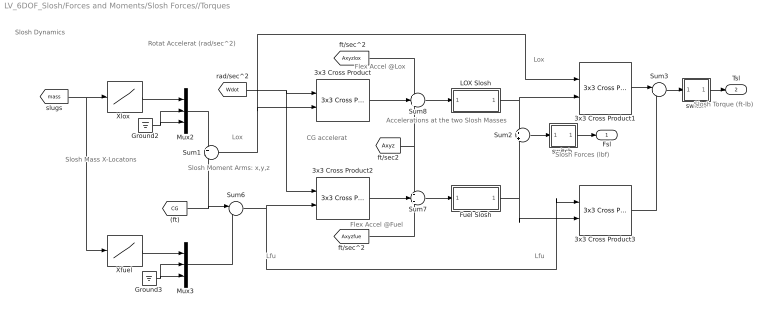
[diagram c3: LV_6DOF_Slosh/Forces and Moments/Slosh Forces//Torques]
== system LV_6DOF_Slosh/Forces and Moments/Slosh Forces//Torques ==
  note: Lfu
  note: Lox
  note: Slosh Torque (ft-lb)
  note: Slosh Forces (lbf)
  note: Slosh Dynamics
  note: Lfu
  note: Accelerations at the two Slosh Masses
  note: Rotat Accelerat (rad/sec^2)
  note: Flex Accel @Lox
  note: CG accelerat
  note: Lox
  note: Slosh Moment Arms: x,y,z
  note: Flex Accel @Fuel
  note: Slosh Mass X-Locatons
  3x3 Cross Product{,1..3} (4 alike) : sharedutil/3x3 Cross Product  aMode=aMode
  Fuel Slosh : Subsystem
  Ground2 : Ground
  Ground3 : Ground
  LOX Slosh : Subsystem
  Mux2 : Mux  Inputs=3
  Mux3 : Mux  Inputs=3
  Sum1 : Sum  Inputs=+|-
  Sum2 : Sum  Inputs=+|+
  Sum3 : Sum  Inputs=|++
  Sum6 : Sum  Inputs=|-+
  Sum7 : Sum  Inputs=+++
  Sum8 : Sum  Inputs=+++
  Xfuel : Lookup  InputValues=Mvsls  Table=Xfuel
  "Xlox " : Lookup  InputValues=Mvsls  Table=Xlox
  switch : Subsystem
  "switch " : Subsystem
  Fsl : Outport
  Tsl : Outport  Port=2
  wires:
  Fuel Slosh/1(Ffuel) -> 3x3 Cross Product3/2, Sum2/2
  3x3 Cross Product1/1 -> Sum3/1
  LOX Slosh/1(Flox) -> 3x3 Cross Product1/2, Sum2/1
  3x3 Cross Product3/1 -> Sum3/2
  Sum3/1 -> switch/1(in)
  Sum2/1 -> "switch "/1(in)
  Sum7/1 -> Fuel Slosh/1(Axyz)
  Sum8/1 -> LOX Slosh/1(Axyz)
  Sum6/1 -> 3x3 Cross Product3/1, 3x3 Cross Product2/2
  3x3 Cross Product/1 -> Sum8/2
  Mux3/1 -> Sum6/2
  [Axyz] -> Sum7/1, Sum8/3
  Mux2/1 -> Sum1/1
  Xfuel/1 -> Mux3/1
  Ground2/1 -> Mux2/2, Mux2/3
  Sum1/1 -> 3x3 Cross Product/2, 3x3 Cross Product1/1
  [mass] -> Xfuel/1, "Xlox "/1
  [CG] -> Sum1/2, Sum6/1
  Ground3/1 -> Mux3/2, Mux3/3
  "Xlox "/1 -> Mux2/1
  [Axyzfue] -> Sum7/3
  [Axyzlox] -> Sum8/1
  [Wdot] -> 3x3 Cross Product2/1, 3x3 Cross Product/1
  3x3 Cross Product2/1 -> Sum7/2
  switch/1(ou) -> Tsl/1
  "switch "/1(ou) -> Fsl/1

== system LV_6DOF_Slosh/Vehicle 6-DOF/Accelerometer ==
  note: CG Accelerat
  note: Moment Arm
  note: Accelerometer Measurement
  note: Rotat accelerat (rad/sec^2)
  note: Translat Accelerat at Gimbal
  note: Accelerations at the Accelerometer and at the Eng. Gimbal
  wdot : Inport
  3x3 Cross Product : sharedutil/3x3 Cross Product  aMode=aMode
  3x3 Cross Product1 : sharedutil/3x3 Cross Product  aMode=aMode
  Accel Loc : Constant  Value=accel
  Gimb 2 CG Mom-Arm : Subsystem
  Memory : Memory  InheritSampleTime=on  LinearizeAsDelay=on
  Sum2 : Sum  Inputs=++|
  Sum3 : Sum  Inputs=-+|
  Sum5 : Sum  Inputs=++|
  "w-dot " : ToWorkspace  VariableName=Wdot  SampleTime=-1
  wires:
  Accel Loc/1 -> Sum3/2
  [CG] -> Sum3/1
  Sum3/1 -> 3x3 Cross Product/2
  3x3 Cross Product/1 -> Sum5/2
  Sum5/1 -> [Axlrm]
  Gimb 2 CG Mom-Arm/1(Lg) -> 3x3 Cross Product1/2
  wdot/1 -> 3x3 Cross Product/1, "w-dot "/1, 3x3 Cross Product1/1, [Wdot]
  [Axyz] -> Sum2/1, Sum5/1
  Sum2/1 -> Memory/1
  3x3 Cross Product1/1 -> Sum2/2
  Memory/1 -> [AxyzGmb]

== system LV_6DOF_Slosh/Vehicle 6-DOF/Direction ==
  note: Direction, Gamma, CrossRange, DownRange
  Ve : Inport
  " " : Integrator
  East : ToWorkspace  VariableName=east  SampleTime=-1
  Heading : ToWorkspace  VariableName=direct  SampleTime=-1
  Int1 : Integrator
  Int2 : Integrator
  North : ToWorkspace  VariableName=north  SampleTime=-1
  Subsystem : Subsystem
  Vearth : ToWorkspace  VariableName=Ve  SampleTime=-1
  Vx : Selector  InputPortWidth=3  IndexOptions=Index vector (dialog)  Indices=[1]  OutputSizes=1
  Vy : Selector  InputPortWidth=3  IndexOptions=Index vector (dialog)  Indices=[2]  OutputSizes=1
  atan1 : Trigonometry  Operator=atan2
  downrange : ToWorkspace  VariableName=dnr  SampleTime=-1
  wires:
  Vx/1 -> atan1/2, Subsystem/1(Vx), Int2/1
  Ve/1 -> Vy/1, Vx/1, Vearth/1
  Vy/1 -> Subsystem/2(Vy), Int1/1, atan1/1
  atan1/1 -> [direct], Heading/1
  Int1/1 -> East/1
  Int2/1 -> North/1
  Subsystem/1(Vxy) -> " "/1
  " "/1 -> downrange/1

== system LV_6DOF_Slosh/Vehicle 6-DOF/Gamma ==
  note: Gamma Angle
  Vecef : Inport
  Recef : Inport  Port=2
  Constant : Constant  Value=1.0e-10
  Divide1 : Product  Inputs=*/
  Dot Product : DotProduct  SaturateOnIntegerOverflow=on
  Dot Product1 : DotProduct  SaturateOnIntegerOverflow=on
  Dot Product3 : DotProduct  SaturateOnIntegerOverflow=on
  Gamma Reference : Subsystem  Tag=STV Subsys  LoadFcn=sigbuilder_block('load');  StartFcn=sigbuilder_block('start');  StopFcn=sigbuilder_block('stop');  ClipboardFcn=sigbuilder_block('clipboard');  mask(Sigbuilder block){tuvar=[0:10]}
      mask help: Sigbuilder GUI
      mask init:
      | if ~strcmp(get_param(bdroot(gcbh),'SimulationStatus'),'stopped') tuvar = sigbuilder_block('maskInit'); end
  Product4 : Product
  Sum1 : Sum  Inputs=|++
  Sum4 : Sum  Inputs=+|-
  Trigonometric Function : Trigonometry  Operator=asin
  V : Math  Operator=sqrt
  V2 : Math  Operator=sqrt
  gama_cmd : ToWorkspace  VariableName=gamacm  SampleTime=-1
  gama_error : ToWorkspace  VariableName=gamerr  SampleTime=-1
  gama_veh : ToWorkspace  VariableName=gama  SampleTime=-1
  r2d : Gain  Gain=r2d
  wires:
  Sum4/1 -> gama_error/1
  Gamma Reference/1(Gama_cmd) -> gama_cmd/1, Sum4/1
  Constant/1 -> Sum1/2
  Product4/1 -> Sum1/1  "XV"
  Dot Product3/1 -> Divide1/1  "X.V"
  Dot Product/1 -> V/1
  Dot Product1/1 -> V2/1
  V/1 -> Product4/2  "X"
  Vecef/1 -> Dot Product1/1, Dot Product1/2, [Vecef], Dot Product3/2
  Trigonometric Function/1 -> r2d/1
  V2/1 -> Product4/1  "V"
  Divide1/1 -> Trigonometric Function/1
  Recef/1 -> Dot Product/2, [Recef], Dot Product3/1, Dot Product/1
  r2d/1 -> gama_veh/1, Sum4/2
  Sum1/1 -> Divide1/2

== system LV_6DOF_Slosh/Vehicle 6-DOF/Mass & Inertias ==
  note: Mass Properties Versus Time
  note: Moments of Inertia Matrix
  Create Moments of Inertia Matrix : sharedutil/Create 3x3 Matrix  aMode=aMode
  Mass Variation : Subsystem
  Moments of Inertia : Subsystem
  mass : Outport
  Inert : Outport  Port=2
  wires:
  Mass Variation/1(mass (slug)) -> mass/1, Moments of Inertia/1(mass)
  Create Moments of Inertia Matrix/1 -> Inert/1
  Moments of Inertia/6(Iyz) -> Create Moments of Inertia Matrix/6, Create Moments of Inertia Matrix/8
  Moments of Inertia/5(Ixz) -> Create Moments of Inertia Matrix/7, Create Moments of Inertia Matrix/3
  Moments of Inertia/2(Iyy) -> Create Moments of Inertia Matrix/5
  Moments of Inertia/3(Izz) -> Create Moments of Inertia Matrix/9
  Moments of Inertia/1(Ixx) -> Create Moments of Inertia Matrix/1
  Moments of Inertia/4(Ixy) -> Create Moments of Inertia Matrix/4, Create Moments of Inertia Matrix/2

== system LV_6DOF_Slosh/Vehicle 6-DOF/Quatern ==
  note: Euler Angles
  in : Inport
  Demux1 : Demux  Outputs=3
  Demux2 : Demux  Outputs=3
  Mux : Mux  Inputs=3
  Rotation Angles to Quaternions : sharedtransform/Rotation Angles to Quaternions  rotationOrder=ZYX  aMode=aMode
  "Theta " : ToWorkspace  VariableName=thet  SampleTime=-1
  roll : ToWorkspace  VariableName=phi  SampleTime=-1
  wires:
  Demux2/2 -> "Theta "/1, [theta3]
  in/1 -> Demux1/1, Demux2/1
  Demux2/3 -> [psi3]
  Demux2/1 -> roll/1, [phi3]
  Rotation Angles to Quaternions/1 -> [qtb2]
  Mux/1 -> Rotation Angles to Quaternions/1
  Demux1/1 -> Mux/3
  Demux1/3 -> Mux/1
  Demux1/2 -> Mux/2

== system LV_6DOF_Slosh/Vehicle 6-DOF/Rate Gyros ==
  note: Rate Integrals
  note: Rate Gyro Measurement
  note: Quaternion Integration
  note: Body Rates
  note: Body Rates
  wrb : Inport
  Attitude : ToWorkspace  VariableName=Euler  SampleTime=-1
  Demux2 : Demux  Outputs=3
  Demux3 : Demux  Outputs=3
  Mux : Mux  Inputs=3
  Mux2 : Mux  Inputs=3
  Pitch Command : Subsystem  Tag=STV Subsys  LoadFcn=sigbuilder_block('load');  StartFcn=sigbuilder_block('start');  StopFcn=sigbuilder_block('stop');  ClipboardFcn=sigbuilder_block('clipboard');  mask(Sigbuilder block){tuvar=[0:10]}
      mask help: Sigbuilder GUI
      mask init:
      | if ~strcmp(get_param(bdroot(gcbh),'SimulationStatus'),'stopped') tuvar = sigbuilder_block('maskInit'); end
  Q-init : Integrator  InitialCondition="[0  -0.70710678118   0   0.70710678118]"  UpperSaturationLimit=628  LowerSaturationLimit=-628
  Quaternion Derivative : MATLAB Function  TreatAsAtomicUnit=on
  Quaternions to Rotation Angles2 : sharedtransform/Quaternions to Rotation Angles  rotationOrder=ZYX  aMode=aMode
  int : Integrator  InitialCondition=Euler_0
  ptch gyro : TransferFcn  Numerator=[100]  Denominator=[1 100]
  roll gyro : TransferFcn  Numerator=[100]  Denominator=[1 100]
  the_cmd : ToWorkspace  VariableName=thec  SampleTime=-1
  theta_body : ToWorkspace  VariableName=theb  SampleTime=-1
  w-body : ToWorkspace  VariableName=Wb  SampleTime=-1
  yaw gyro : TransferFcn  Numerator=[100]  Denominator=[1 100]
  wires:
  int/1 -> Demux2/1
  Demux2/3 -> [psib]
  Demux2/1 -> [phib]
  Demux2/2 -> theta_body/1, [thetab]
  Mux2/1 -> Quaternion Derivative/2(wb)
  Q-init/1 -> Quaternion Derivative/1(qi), Quaternions to Rotation Angles2/1, [qtb3]
  Demux3/3 -> yaw gyro/1, Mux2/3  "R"
  Demux3/1 -> roll gyro/1, Mux2/1  "P"
  Demux3/2 -> ptch gyro/1, Mux2/2  "Q"
  Mux/1 -> [Gyros]
  Quaternion Derivative/1(Qd) -> Q-init/1
  roll gyro/1 -> Mux/1
  ptch gyro/1 -> Mux/2
  yaw gyro/1 -> Mux/3
  Quaternions to Rotation Angles2/1 -> Attitude/1
  wrb/1 -> Demux3/1, w-body/1, int/1
  Pitch Command/1(Theta_cmd) -> the_cmd/1

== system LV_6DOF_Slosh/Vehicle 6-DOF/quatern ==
  in1 : Inport
  in : Inport  Port=2
  Direction Cosine Matrix to Quaternions : sharedtransform/Direction Cosine Matrix  to Quaternions  aMode=0  action=None  tolerance=eps(2)
  Scope : Scope
  ecf 2 geo1 : Product  Multiplication=Matrix(*)
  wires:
  in/1 -> ecf 2 geo1/1, [DCM], Direction Cosine Matrix to Quaternions/1
  Direction Cosine Matrix to Quaternions/1 -> [qtb]
  in1/1 -> ecf 2 geo1/2
  ecf 2 geo1/1 -> Scope/1

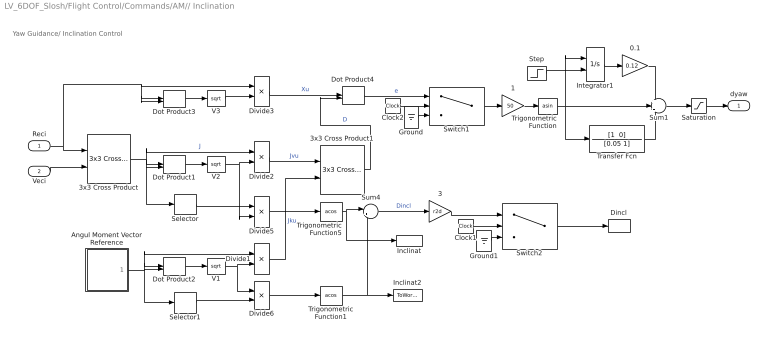
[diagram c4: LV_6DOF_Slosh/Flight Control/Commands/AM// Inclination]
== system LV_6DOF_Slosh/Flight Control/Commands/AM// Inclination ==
  note: Yaw Guidance/ Inclination Control
  Reci : Inport
  Veci : Inport  Port=2
  0.1 : Gain  Gain=0.12
  1 : Gain  Gain=50
  3 : Gain  Gain=r2d
  3x3 Cross Product : sharedutil/3x3 Cross Product  aMode=aMode
  3x3 Cross Product1 : sharedutil/3x3 Cross Product  aMode=aMode
  Angul Moment Vector Reference : Subsystem
  Clock1 : Clock
  Clock2 : Clock
  Dincl : ToWorkspace  VariableName=Dincl  SampleTime=-1
  Divide{1..3,5} (4 alike) : Product  Inputs=*/
  Divide6 : Product  Inputs=/*
  Dot Product{1..4} (4 alike) : DotProduct  SaturateOnIntegerOverflow=on
  Ground : Ground
  Ground1 : Ground
  Inclinat : ToWorkspace  VariableName=Inclin  SampleTime=-1
  Inclinat2 : ToWorkspace  VariableName=Inclin2  SampleTime=-1
  Integrator1 : Integrator  ExternalReset=rising
  Saturation : Saturate  UpperLimit=0.05  LowerLimit=-0.05
  Selector : Selector  InputPortWidth=3  IndexOptions=Index vector (dialog)  Indices=[3]  OutputSizes=1
  Selector1 : Selector  InputPortWidth=3  IndexOptions=Index vector (dialog)  Indices=[3]  OutputSizes=1
  Step : Step  Time=T3b  SampleTime=0
  Sum1 : Sum  Inputs=+++
  Sum4 : Sum  Inputs=|+-
  Switch1 : Switch  Criteria=u2 > Threshold  Threshold=T3b
  Switch2 : Switch  Criteria=u2 > Threshold  Threshold=T3b
  Transfer Fcn : TransferFcn  Numerator="[1  0]"  Denominator=[0.05 1]
  Trigonometric Function : Trigonometry  Operator=asin
  Trigonometric Function1 : Trigonometry  Operator=acos
  Trigonometric Function5 : Trigonometry  Operator=acos
  V1 : Math  Operator=sqrt
  V2 : Math  Operator=sqrt
  V3 : Math  Operator=sqrt
  dyaw : Outport
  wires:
  Sum1/1 -> Saturation/1
  Saturation/1 -> dyaw/1
  Switch1/1 -> 1/1
  0.1/1 -> Sum1/1
  Transfer Fcn/1 -> Sum1/3
  Integrator1/1 -> 0.1/1
  Step/1 -> Integrator1/2
  Switch2/1 -> Dincl/1
  3/1 -> Switch2/1
  1/1 -> Trigonometric Function/1
  Trigonometric Function/1 -> Sum1/2, Transfer Fcn/1, Integrator1/1
  Angul Moment Vector Reference/1(J3) -> Dot Product2/1, Divide1/1, Dot Product2/2, Selector1/1
  Trigonometric Function1/1 -> Inclinat2/1, Sum4/2
  Trigonometric Function5/1 -> Inclinat/1, Sum4/1
  Sum4/1 -> 3/1  "Dincl"
  Clock1/1 -> Switch2/2
  Ground1/1 -> Switch2/3
  Divide6/1 -> Trigonometric Function1/1
  Divide5/1 -> Trigonometric Function5/1
  Selector1/1 -> Divide6/2
  Selector/1 -> Divide5/1
  Dot Product4/1 -> Switch1/1  "e"
  Ground/1 -> Switch1/3
  Clock2/1 -> Switch1/2
  3x3 Cross Product1/1 -> Dot Product4/2  "D"
  Divide3/1 -> Dot Product4/1  "Xu"
  V3/1 -> Divide3/2
  Dot Product3/1 -> V3/1
  Divide2/1 -> 3x3 Cross Product1/1  "Jvu"
  V2/1 -> Divide2/2, Divide5/2
  Dot Product1/1 -> V2/1
  Divide1/1 -> 3x3 Cross Product1/2  "Jku"
  V1/1 -> Divide1/2, Divide6/1
  Dot Product2/1 -> V1/1
  Reci/1 -> 3x3 Cross Product/1, Divide3/1, Dot Product3/1, Dot Product3/2
  3x3 Cross Product/1 -> Dot Product1/1, Dot Product1/2, Selector/1, Divide2/1  "J"
  Veci/1 -> 3x3 Cross Product/2
